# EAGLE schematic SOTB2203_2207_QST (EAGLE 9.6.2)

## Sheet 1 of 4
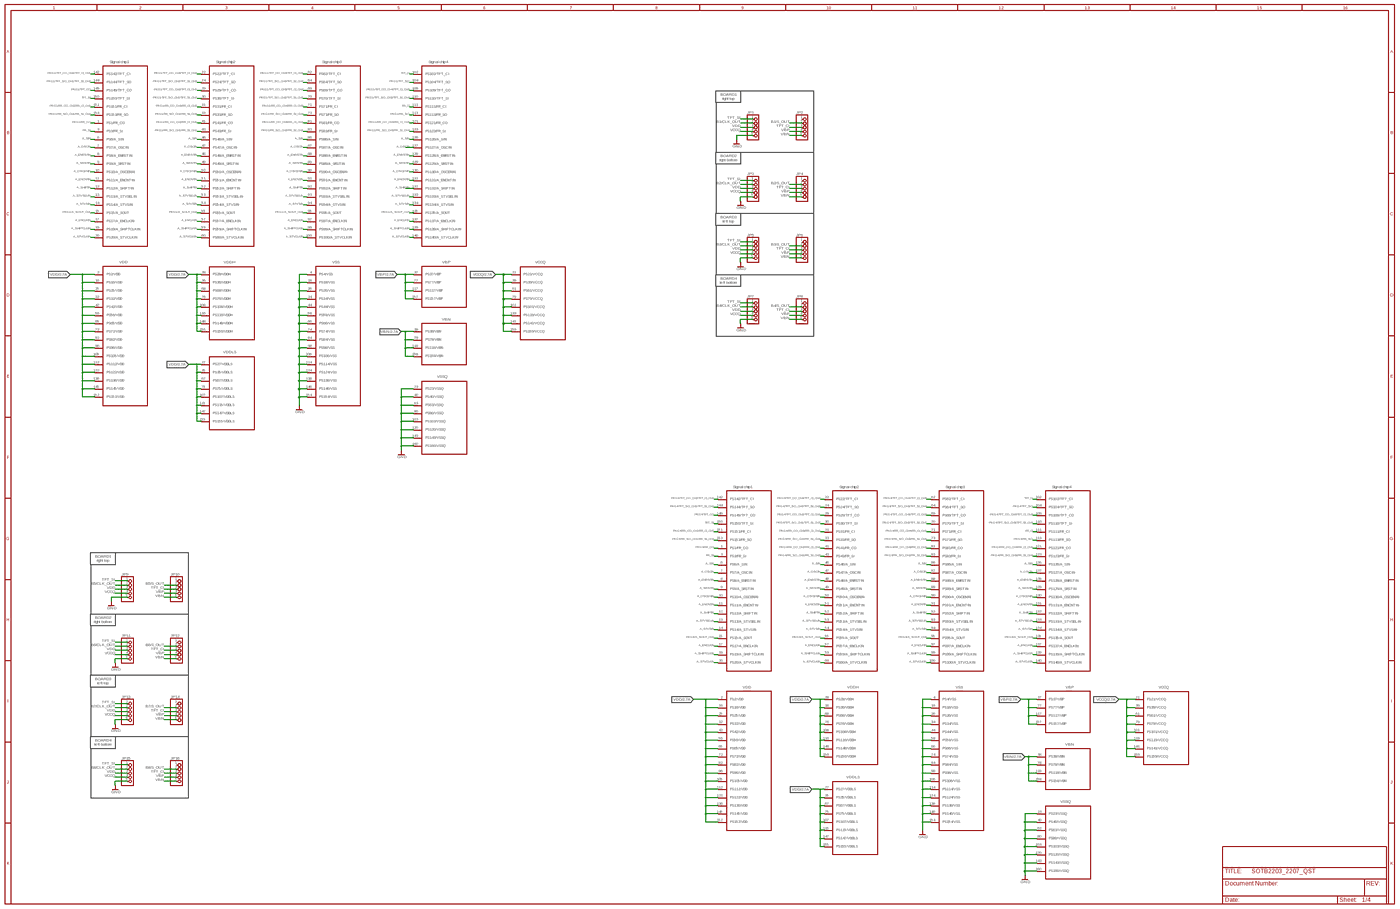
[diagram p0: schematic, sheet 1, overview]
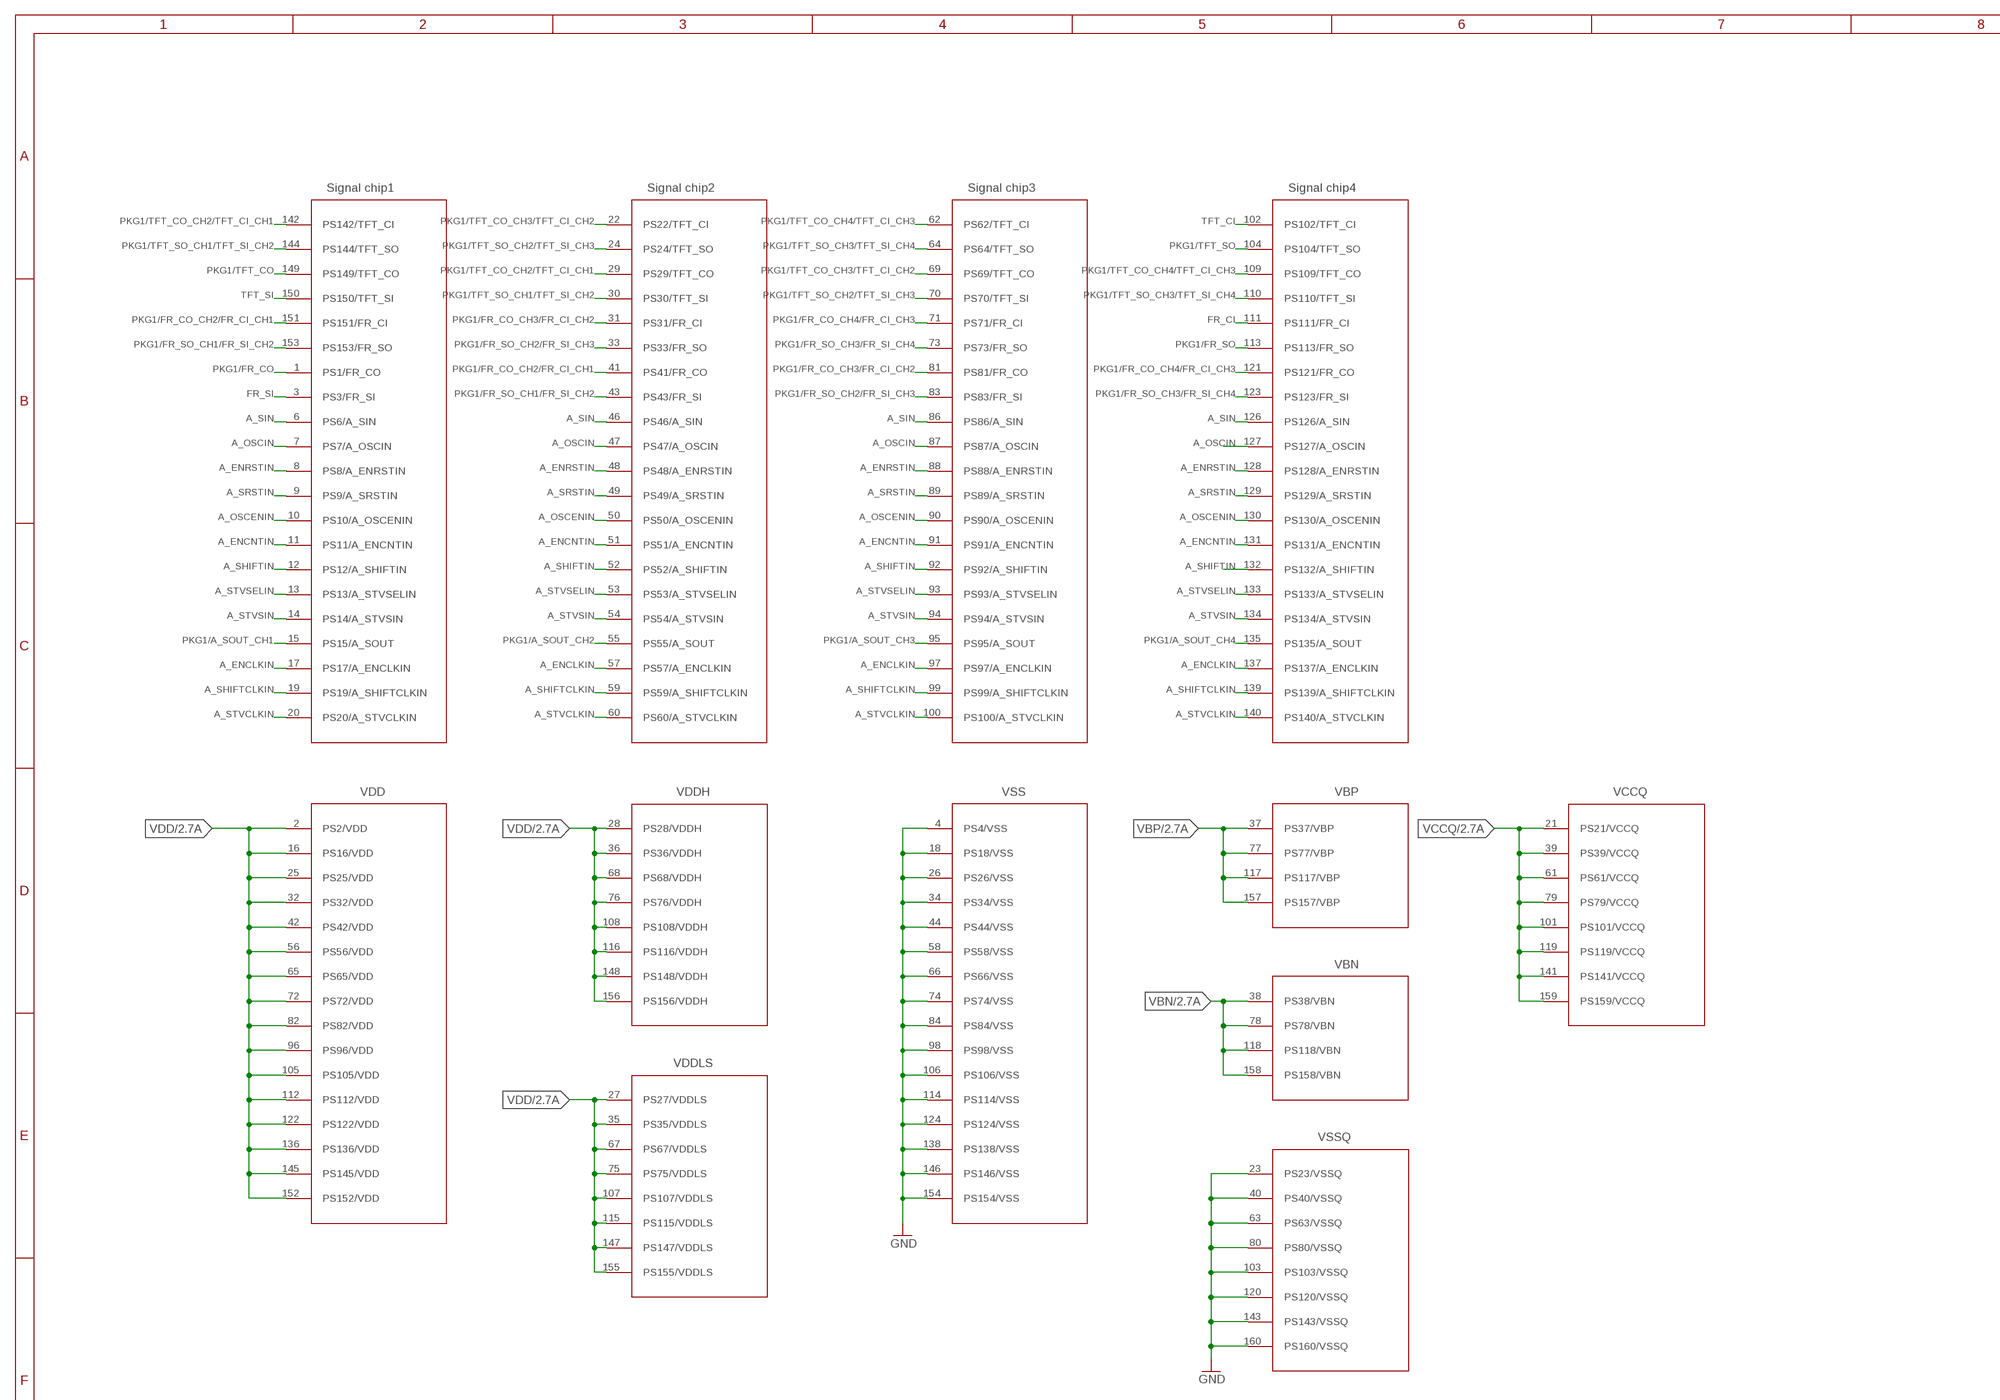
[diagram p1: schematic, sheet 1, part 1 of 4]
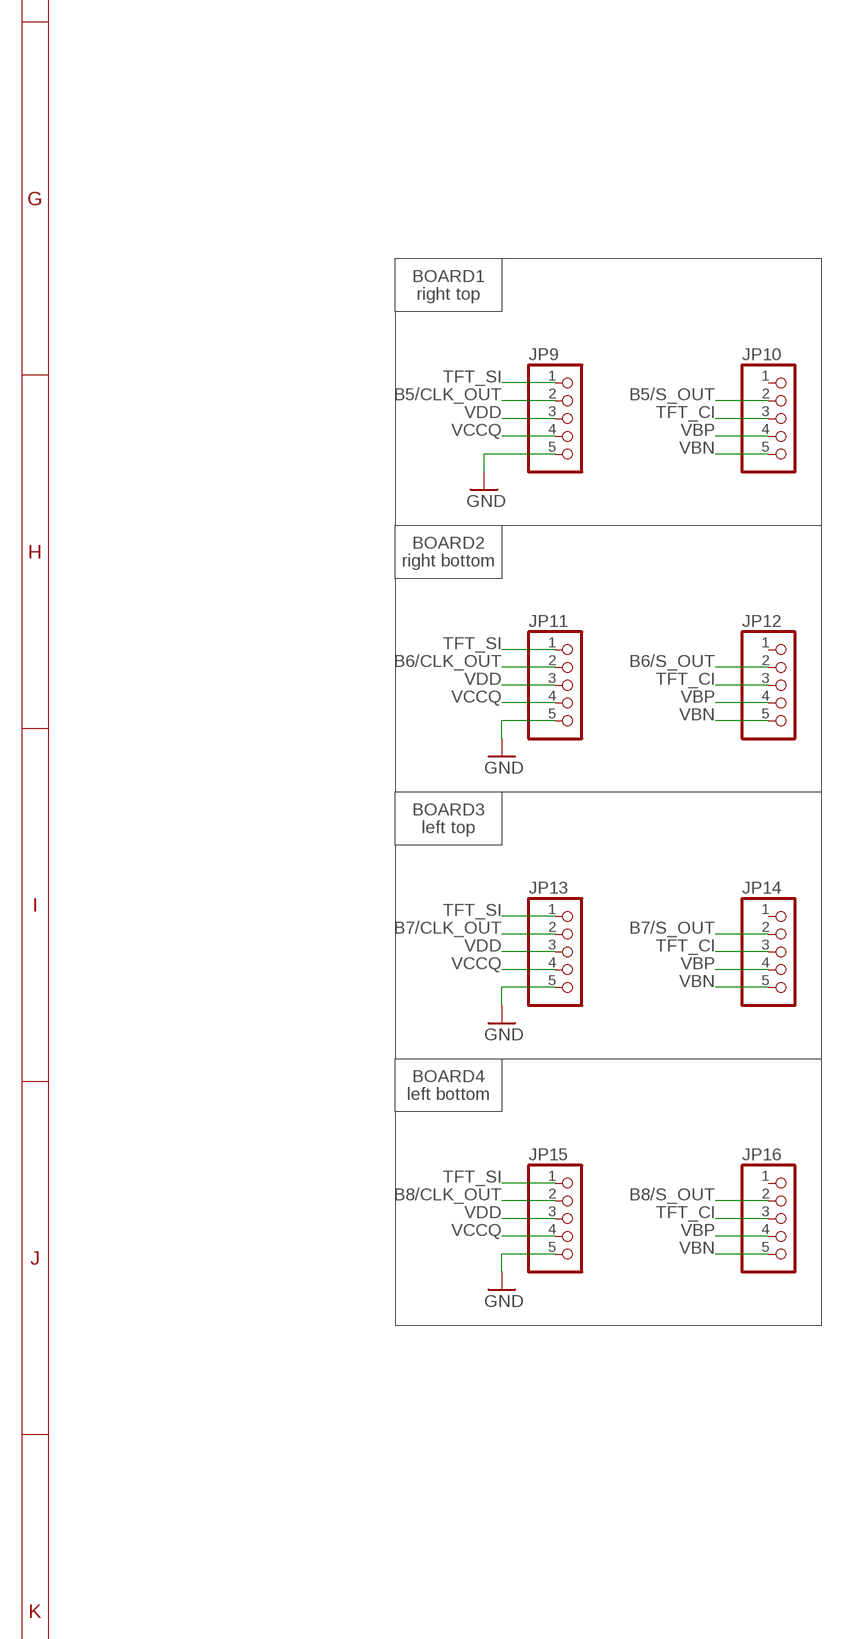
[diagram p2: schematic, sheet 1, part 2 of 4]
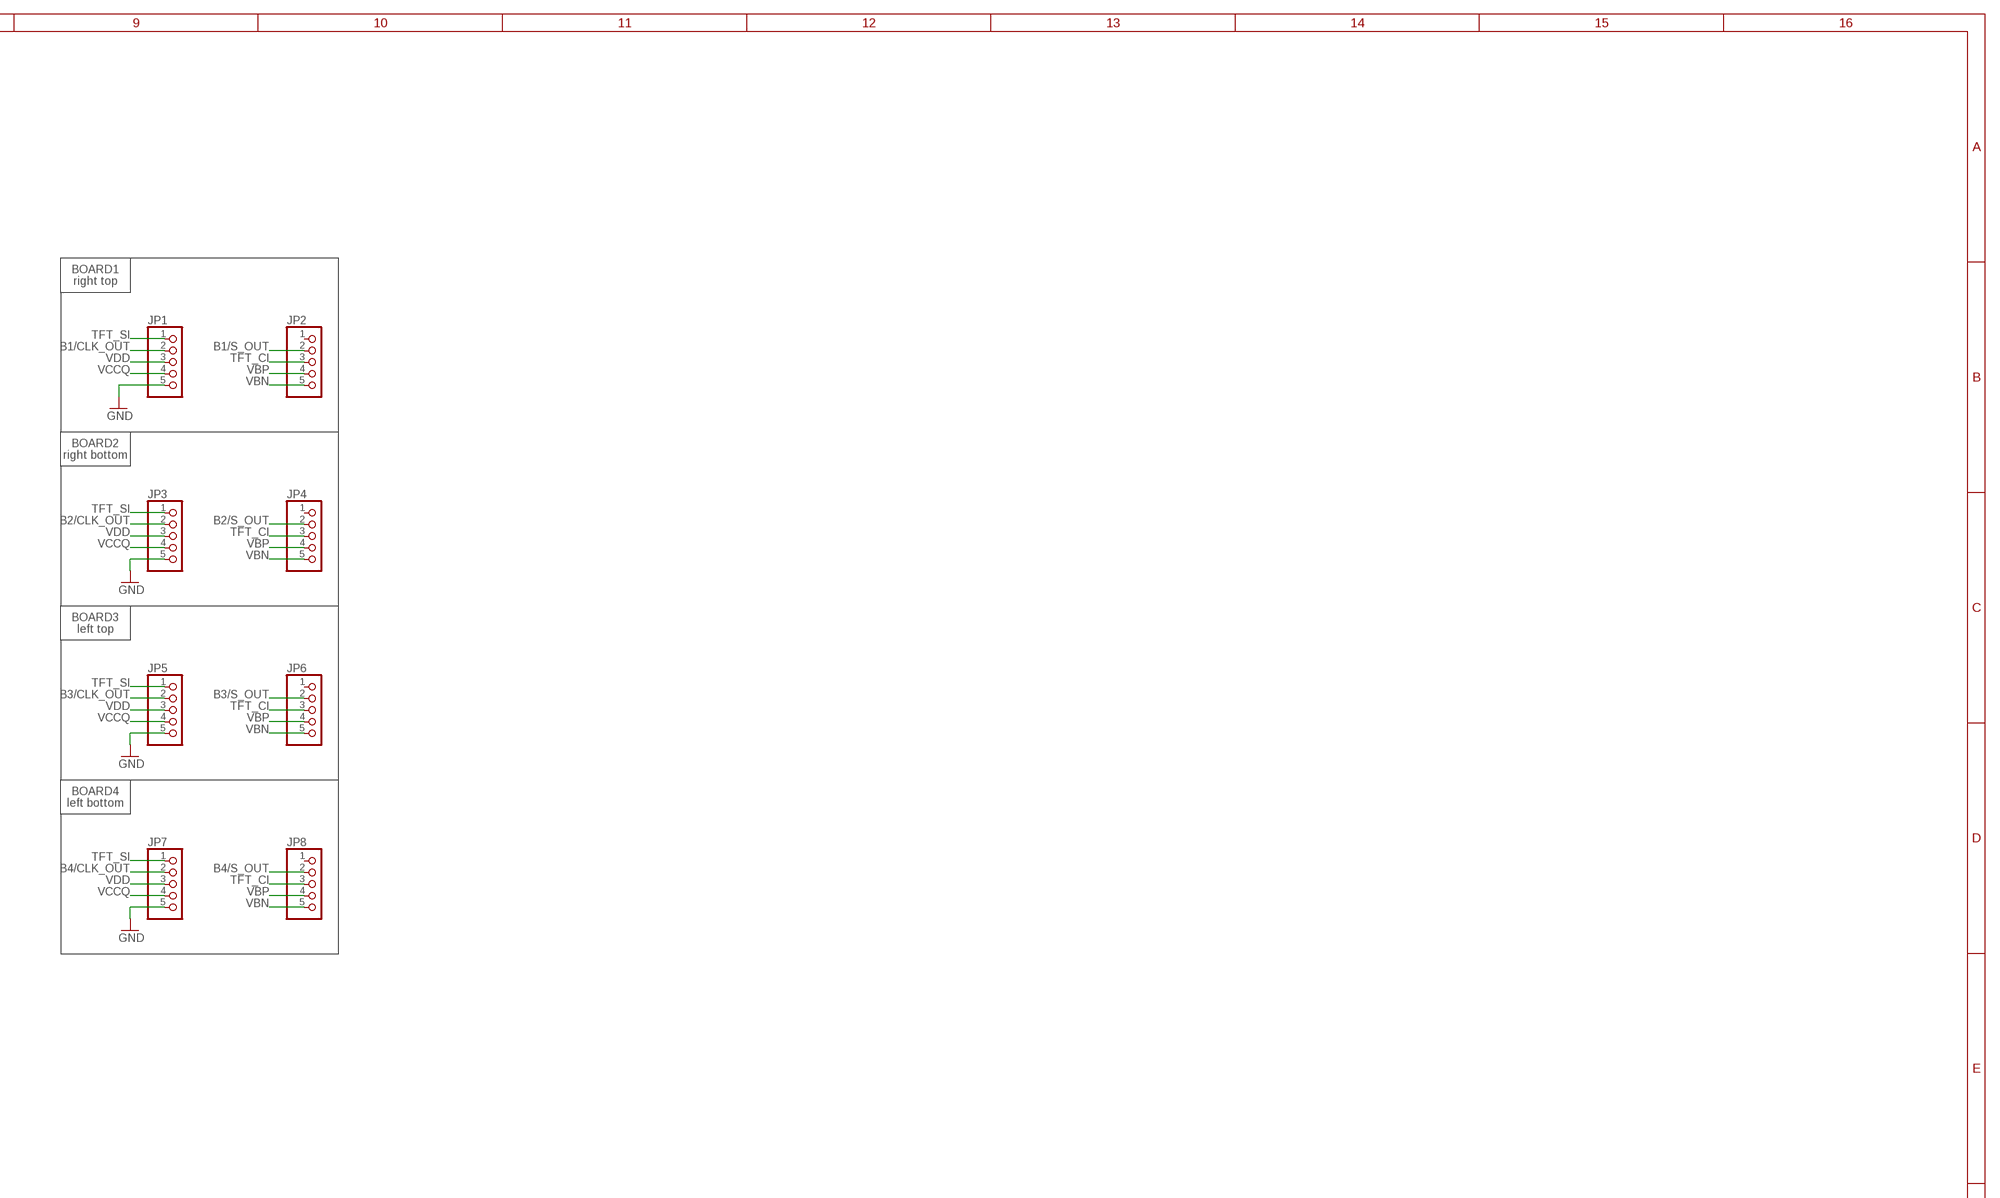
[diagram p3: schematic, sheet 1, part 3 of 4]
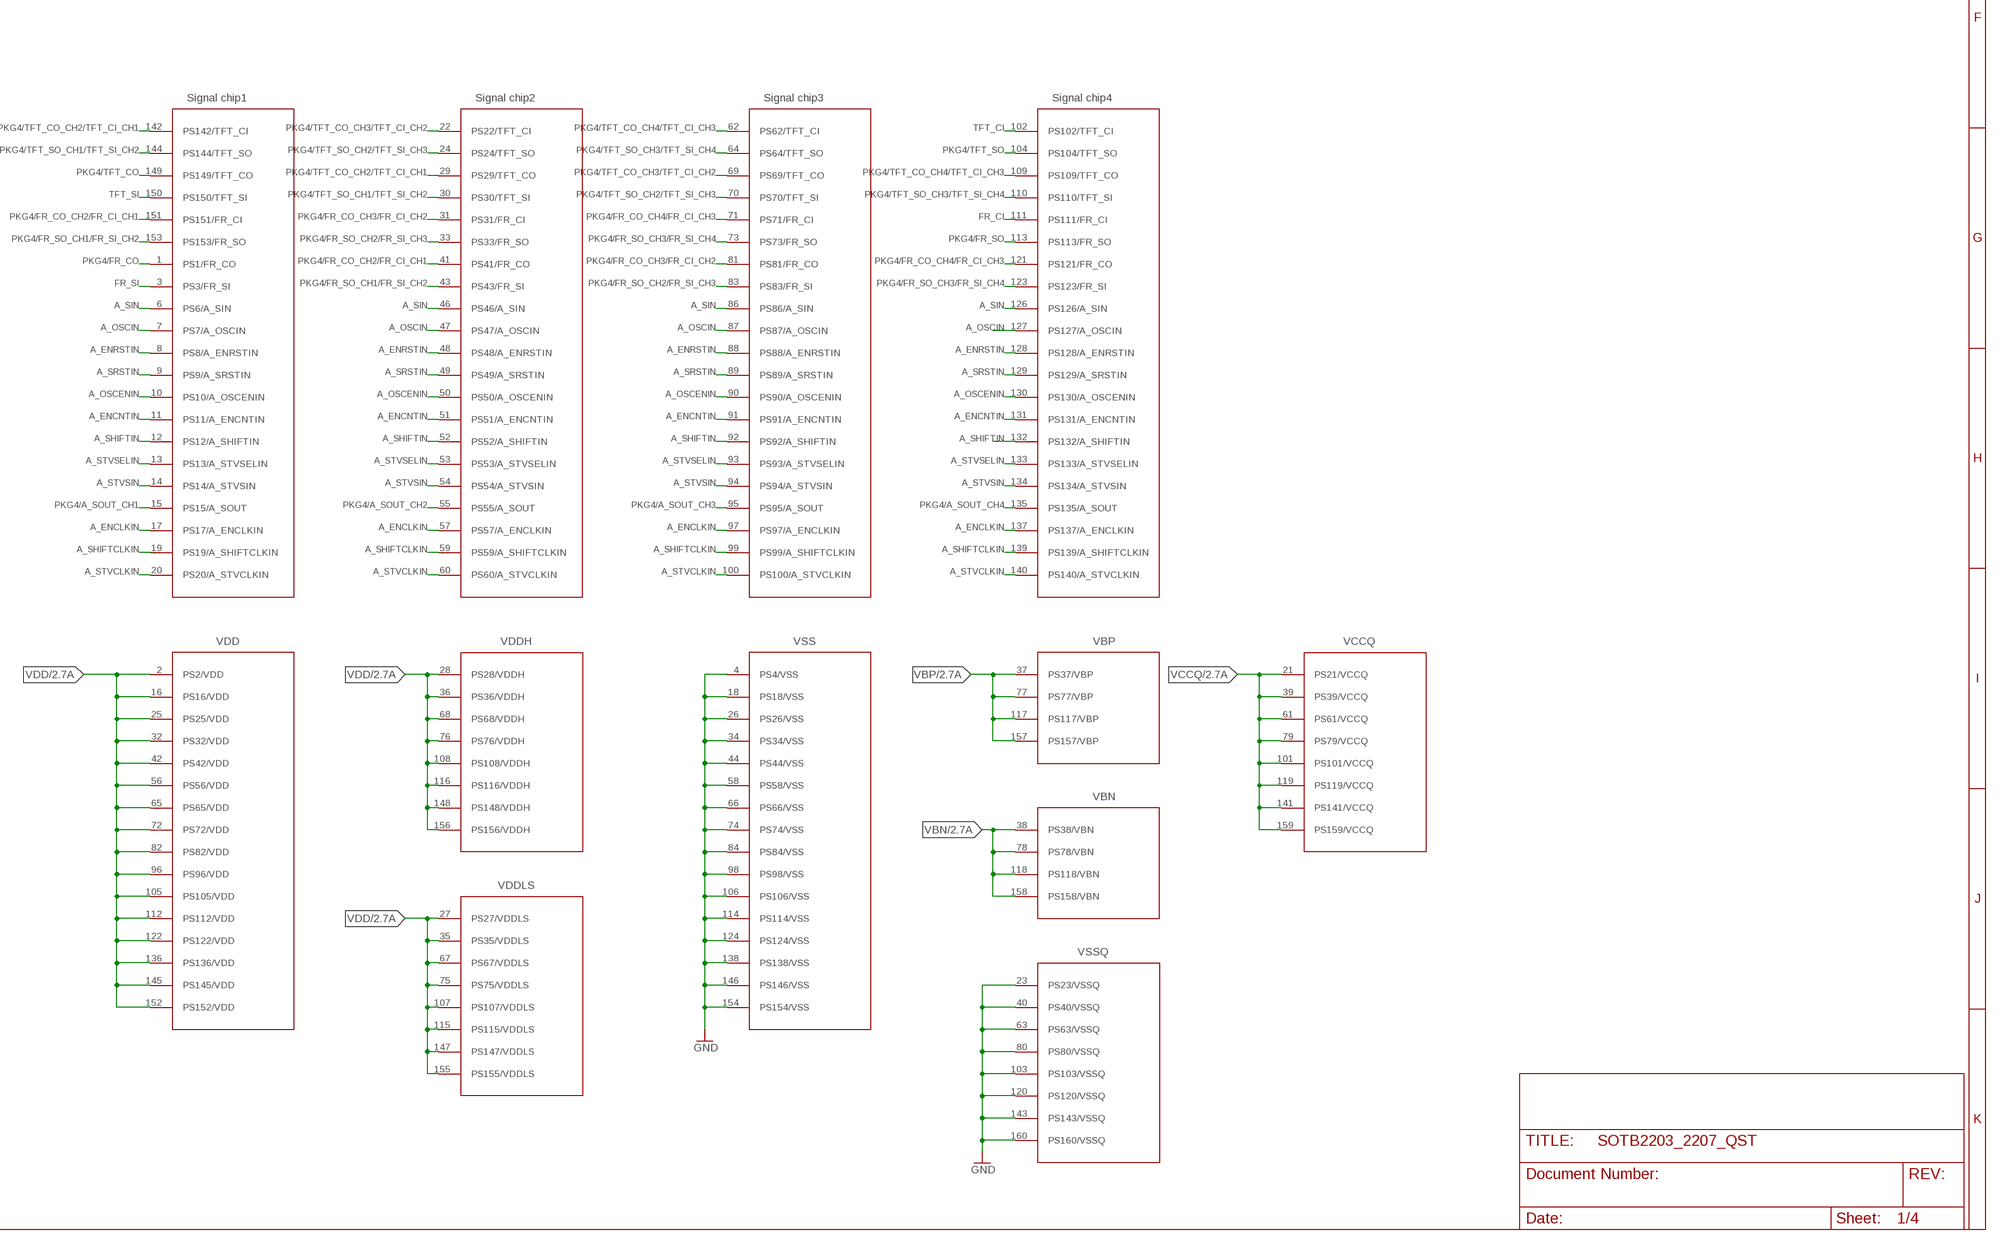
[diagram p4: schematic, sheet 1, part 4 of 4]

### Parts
JP1  PINHD-1X5  [1X05]
JP2  PINHD-1X5  [1X05]
JP3  PINHD-1X5  [1X05]
JP4  PINHD-1X5  [1X05]
JP5  PINHD-1X5  [1X05]
JP6  PINHD-1X5  [1X05]
JP7  PINHD-1X5  [1X05]
JP8  PINHD-1X5  [1X05]
JP9  PINHD-1X5  [1X05]
JP10  PINHD-1X5  [1X05]
JP11  PINHD-1X5  [1X05]
JP12  PINHD-1X5  [1X05]
JP13  PINHD-1X5  [1X05]
JP14  PINHD-1X5  [1X05]
JP15  PINHD-1X5  [1X05]
JP16  PINHD-1X5  [1X05]
PKG1  SOTB2207_4CHIP  [IC149-160-123-B5]
PKG4  SOTB2207_4CHIP  [IC149-160-123-B5]

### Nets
A_ENCLKIN: PKG1.17(PS17/A_ENCLKIN) PKG1.57(PS57/A_ENCLKIN) PKG1.97(PS97/A_ENCLKIN) PKG1.137(PS137/A_ENCLKIN) PKG4.17(PS17/A_ENCLKIN) PKG4.57(PS57/A_ENCLKIN) PKG4.97(PS97/A_ENCLKIN) PKG4.137(PS137/A_ENCLKIN) ; also sheet 2,4
A_ENCNTIN: PKG1.11(PS11/A_ENCNTIN) PKG1.51(PS51/A_ENCNTIN) PKG1.91(PS91/A_ENCNTIN) PKG1.131(PS131/A_ENCNTIN) PKG4.11(PS11/A_ENCNTIN) PKG4.51(PS51/A_ENCNTIN) PKG4.91(PS91/A_ENCNTIN) PKG4.131(PS131/A_ENCNTIN) ; also sheet 2,4
A_ENRSTIN: PKG1.8(PS8/A_ENRSTIN) PKG1.48(PS48/A_ENRSTIN) PKG1.88(PS88/A_ENRSTIN) PKG1.128(PS128/A_ENRSTIN) PKG4.8(PS8/A_ENRSTIN) PKG4.48(PS48/A_ENRSTIN) PKG4.88(PS88/A_ENRSTIN) PKG4.128(PS128/A_ENRSTIN) ; also sheet 2,4
A_OSCENIN: PKG1.10(PS10/A_OSCENIN) PKG1.50(PS50/A_OSCENIN) PKG1.90(PS90/A_OSCENIN) PKG1.130(PS130/A_OSCENIN) PKG4.10(PS10/A_OSCENIN) PKG4.50(PS50/A_OSCENIN) PKG4.90(PS90/A_OSCENIN) PKG4.130(PS130/A_OSCENIN) ; also sheet 2,4
A_OSCIN: PKG1.7(PS7/A_OSCIN) PKG1.47(PS47/A_OSCIN) PKG1.87(PS87/A_OSCIN) PKG1.127(PS127/A_OSCIN) PKG4.7(PS7/A_OSCIN) PKG4.47(PS47/A_OSCIN) PKG4.87(PS87/A_OSCIN) PKG4.127(PS127/A_OSCIN) ; also sheet 2,4
A_SHIFTCLKIN: PKG1.19(PS19/A_SHIFTCLKIN) PKG1.59(PS59/A_SHIFTCLKIN) PKG1.99(PS99/A_SHIFTCLKIN) PKG1.139(PS139/A_SHIFTCLKIN) PKG4.19(PS19/A_SHIFTCLKIN) PKG4.59(PS59/A_SHIFTCLKIN) PKG4.99(PS99/A_SHIFTCLKIN) PKG4.139(PS139/A_SHIFTCLKIN) ; also sheet 2,4
A_SHIFTIN: PKG1.12(PS12/A_SHIFTIN) PKG1.52(PS52/A_SHIFTIN) PKG1.92(PS92/A_SHIFTIN) PKG1.132(PS132/A_SHIFTIN) PKG4.12(PS12/A_SHIFTIN) PKG4.52(PS52/A_SHIFTIN) PKG4.92(PS92/A_SHIFTIN) PKG4.132(PS132/A_SHIFTIN) ; also sheet 2,4
A_SIN: PKG1.6(PS6/A_SIN) PKG1.46(PS46/A_SIN) PKG1.86(PS86/A_SIN) PKG1.126(PS126/A_SIN) PKG4.6(PS6/A_SIN) PKG4.46(PS46/A_SIN) PKG4.86(PS86/A_SIN) PKG4.126(PS126/A_SIN) ; also sheet 2,4
A_SRSTIN: PKG1.9(PS9/A_SRSTIN) PKG1.49(PS49/A_SRSTIN) PKG1.89(PS89/A_SRSTIN) PKG1.129(PS129/A_SRSTIN) PKG4.9(PS9/A_SRSTIN) PKG4.49(PS49/A_SRSTIN) PKG4.89(PS89/A_SRSTIN) PKG4.129(PS129/A_SRSTIN) ; also sheet 2,4
A_STVCLKIN: PKG1.20(PS20/A_STVCLKIN) PKG1.60(PS60/A_STVCLKIN) PKG1.100(PS100/A_STVCLKIN) PKG1.140(PS140/A_STVCLKIN) PKG4.20(PS20/A_STVCLKIN) PKG4.60(PS60/A_STVCLKIN) PKG4.100(PS100/A_STVCLKIN) PKG4.140(PS140/A_STVCLKIN) ; also sheet 2,4
A_STVSELIN: PKG1.13(PS13/A_STVSELIN) PKG1.53(PS53/A_STVSELIN) PKG1.93(PS93/A_STVSELIN) PKG1.133(PS133/A_STVSELIN) PKG4.13(PS13/A_STVSELIN) PKG4.53(PS53/A_STVSELIN) PKG4.93(PS93/A_STVSELIN) PKG4.133(PS133/A_STVSELIN) ; also sheet 2,4
A_STVSIN: PKG1.14(PS14/A_STVSIN) PKG1.54(PS54/A_STVSIN) PKG1.94(PS94/A_STVSIN) PKG1.134(PS134/A_STVSIN) PKG4.14(PS14/A_STVSIN) PKG4.54(PS54/A_STVSIN) PKG4.94(PS94/A_STVSIN) PKG4.134(PS134/A_STVSIN) ; also sheet 2,4
B1/CLK_OUT: JP1.2 ; also sheet 2,4
B1/S_OUT: JP2.2 ; also sheet 2,4
B2/CLK_OUT: JP3.2 ; also sheet 2,4
B2/S_OUT: JP4.2 ; also sheet 2,4
B3/CLK_OUT: JP5.2 ; also sheet 2,4
B3/S_OUT: JP6.2 ; also sheet 2,4
B4/CLK_OUT: JP7.2 ; also sheet 2,4
B4/S_OUT: JP8.2 ; also sheet 2,4
B5/CLK_OUT: JP9.2 ; also sheet 2,4
B5/S_OUT: JP10.2 ; also sheet 2,4
B6/CLK_OUT: JP11.2 ; also sheet 2,4
B6/S_OUT: JP12.2 ; also sheet 2,4
B7/CLK_OUT: JP13.2 ; also sheet 2,4
B7/S_OUT: JP14.2 ; also sheet 2,4
B8/CLK_OUT: JP15.2 ; also sheet 2,4
B8/S_OUT: JP16.2 ; also sheet 2,4
FR_CI: PKG1.111(PS111/FR_CI) PKG4.111(PS111/FR_CI) ; also sheet 2,4
FR_SI: PKG1.3(PS3/FR_SI) PKG4.3(PS3/FR_SI) ; also sheet 2,4
GND: JP1.5 JP3.5 JP5.5 JP7.5 JP9.5 JP11.5 JP13.5 JP15.5 PKG1.4(PS4/VSS) PKG1.18(PS18/VSS) PKG1.23(PS23/VSSQ) PKG1.26(PS26/VSS) PKG1.34(PS34/VSS) PKG1.40(PS40/VSSQ) PKG1.44(PS44/VSS) PKG1.58(PS58/VSS) PKG1.63(PS63/VSSQ) PKG1.66(PS66/VSS) PKG1.74(PS74/VSS) PKG1.80(PS80/VSSQ) PKG1.84(PS84/VSS) PKG1.98(PS98/VSS) PKG1.103(PS103/VSSQ) PKG1.106(PS106/VSS) PKG1.114(PS114/VSS) PKG1.120(PS120/VSSQ) PKG1.124(PS124/VSS) PKG1.138(PS138/VSS) PKG1.143(PS143/VSSQ) PKG1.146(PS146/VSS) PKG1.154(PS154/VSS) PKG1.160(PS160/VSSQ) PKG4.4(PS4/VSS) PKG4.18(PS18/VSS) PKG4.23(PS23/VSSQ) PKG4.26(PS26/VSS) PKG4.34(PS34/VSS) PKG4.40(PS40/VSSQ) PKG4.44(PS44/VSS) PKG4.58(PS58/VSS) PKG4.63(PS63/VSSQ) PKG4.66(PS66/VSS) PKG4.74(PS74/VSS) PKG4.80(PS80/VSSQ) PKG4.84(PS84/VSS) PKG4.98(PS98/VSS) PKG4.103(PS103/VSSQ) PKG4.106(PS106/VSS) PKG4.114(PS114/VSS) PKG4.120(PS120/VSSQ) PKG4.124(PS124/VSS) PKG4.138(PS138/VSS) PKG4.143(PS143/VSSQ) PKG4.146(PS146/VSS) PKG4.154(PS154/VSS) PKG4.160(PS160/VSSQ) ; also sheet 2,3,4
PKG1/A_SOUT_CH1: PKG1.15(PS15/A_SOUT) ; also sheet 2,4
PKG1/A_SOUT_CH2: PKG1.55(PS55/A_SOUT) ; also sheet 2,4
PKG1/A_SOUT_CH3: PKG1.95(PS95/A_SOUT) ; also sheet 2,4
PKG1/A_SOUT_CH4: PKG1.135(PS135/A_SOUT) ; also sheet 2,4
PKG1/FR_CO: PKG1.1(PS1/FR_CO) ; also sheet 2,4
PKG1/FR_CO_CH2/FR_CI_CH1: PKG1.41(PS41/FR_CO) PKG1.151(PS151/FR_CI)
PKG1/FR_CO_CH3/FR_CI_CH2: PKG1.31(PS31/FR_CI) PKG1.81(PS81/FR_CO)
PKG1/FR_CO_CH4/FR_CI_CH3: PKG1.71(PS71/FR_CI) PKG1.121(PS121/FR_CO)
PKG1/FR_SO: PKG1.113(PS113/FR_SO) ; also sheet 2,4
PKG1/FR_SO_CH1/FR_SI_CH2: PKG1.43(PS43/FR_SI) PKG1.153(PS153/FR_SO)
PKG1/FR_SO_CH2/FR_SI_CH3: PKG1.33(PS33/FR_SO) PKG1.83(PS83/FR_SI)
PKG1/FR_SO_CH3/FR_SI_CH4: PKG1.73(PS73/FR_SO) PKG1.123(PS123/FR_SI)
PKG1/TFT_CO: PKG1.149(PS149/TFT_CO) ; also sheet 2,4
PKG1/TFT_CO_CH2/TFT_CI_CH1: PKG1.29(PS29/TFT_CO) PKG1.142(PS142/TFT_CI)
PKG1/TFT_CO_CH3/TFT_CI_CH2: PKG1.22(PS22/TFT_CI) PKG1.69(PS69/TFT_CO)
PKG1/TFT_CO_CH4/TFT_CI_CH3: PKG1.62(PS62/TFT_CI) PKG1.109(PS109/TFT_CO)
PKG1/TFT_SO: PKG1.104(PS104/TFT_SO) ; also sheet 2,4
PKG1/TFT_SO_CH1/TFT_SI_CH2: PKG1.30(PS30/TFT_SI) PKG1.144(PS144/TFT_SO)
PKG1/TFT_SO_CH2/TFT_SI_CH3: PKG1.24(PS24/TFT_SO) PKG1.70(PS70/TFT_SI)
PKG1/TFT_SO_CH3/TFT_SI_CH4: PKG1.64(PS64/TFT_SO) PKG1.110(PS110/TFT_SI)
PKG4/A_SOUT_CH1: PKG4.15(PS15/A_SOUT) ; also sheet 2,4
PKG4/A_SOUT_CH2: PKG4.55(PS55/A_SOUT) ; also sheet 2,4
PKG4/A_SOUT_CH3: PKG4.95(PS95/A_SOUT) ; also sheet 2,4
PKG4/A_SOUT_CH4: PKG4.135(PS135/A_SOUT) ; also sheet 2,4
PKG4/FR_CO: PKG4.1(PS1/FR_CO) ; also sheet 2,4
PKG4/FR_CO_CH2/FR_CI_CH1: PKG4.41(PS41/FR_CO) PKG4.151(PS151/FR_CI)
PKG4/FR_CO_CH3/FR_CI_CH2: PKG4.31(PS31/FR_CI) PKG4.81(PS81/FR_CO)
PKG4/FR_CO_CH4/FR_CI_CH3: PKG4.71(PS71/FR_CI) PKG4.121(PS121/FR_CO)
PKG4/FR_SO: PKG4.113(PS113/FR_SO) ; also sheet 2,4
PKG4/FR_SO_CH1/FR_SI_CH2: PKG4.43(PS43/FR_SI) PKG4.153(PS153/FR_SO)
PKG4/FR_SO_CH2/FR_SI_CH3: PKG4.33(PS33/FR_SO) PKG4.83(PS83/FR_SI)
PKG4/FR_SO_CH3/FR_SI_CH4: PKG4.73(PS73/FR_SO) PKG4.123(PS123/FR_SI)
PKG4/TFT_CO: PKG4.149(PS149/TFT_CO) ; also sheet 2,4
PKG4/TFT_CO_CH2/TFT_CI_CH1: PKG4.29(PS29/TFT_CO) PKG4.142(PS142/TFT_CI)
PKG4/TFT_CO_CH3/TFT_CI_CH2: PKG4.22(PS22/TFT_CI) PKG4.69(PS69/TFT_CO)
PKG4/TFT_CO_CH4/TFT_CI_CH3: PKG4.62(PS62/TFT_CI) PKG4.109(PS109/TFT_CO)
PKG4/TFT_SO: PKG4.104(PS104/TFT_SO) ; also sheet 2,4
PKG4/TFT_SO_CH1/TFT_SI_CH2: PKG4.30(PS30/TFT_SI) PKG4.144(PS144/TFT_SO)
PKG4/TFT_SO_CH2/TFT_SI_CH3: PKG4.24(PS24/TFT_SO) PKG4.70(PS70/TFT_SI)
PKG4/TFT_SO_CH3/TFT_SI_CH4: PKG4.64(PS64/TFT_SO) PKG4.110(PS110/TFT_SI)
TFT_CI: JP2.3 JP4.3 JP6.3 JP8.3 JP10.3 JP12.3 JP14.3 JP16.3 PKG1.102(PS102/TFT_CI) PKG4.102(PS102/TFT_CI) ; also sheet 2,4
TFT_SI: JP1.1 JP3.1 JP5.1 JP7.1 JP9.1 JP11.1 JP13.1 JP15.1 PKG1.150(PS150/TFT_SI) PKG4.150(PS150/TFT_SI) ; also sheet 2,4
VBN: JP2.5 JP4.5 JP6.5 JP8.5 JP10.5 JP12.5 JP14.5 JP16.5 PKG1.38(PS38/VBN) PKG1.78(PS78/VBN) PKG1.118(PS118/VBN) PKG1.158(PS158/VBN) PKG4.38(PS38/VBN) PKG4.78(PS78/VBN) PKG4.118(PS118/VBN) PKG4.158(PS158/VBN) ; also sheet 2,3,4
VBP: JP2.4 JP4.4 JP6.4 JP8.4 JP10.4 JP12.4 JP14.4 JP16.4 PKG1.37(PS37/VBP) PKG1.77(PS77/VBP) PKG1.117(PS117/VBP) PKG1.157(PS157/VBP) PKG4.37(PS37/VBP) PKG4.77(PS77/VBP) PKG4.117(PS117/VBP) PKG4.157(PS157/VBP) ; also sheet 2,3,4
VCCQ: JP1.4 JP3.4 JP5.4 JP7.4 JP9.4 JP11.4 JP13.4 JP15.4 PKG1.21(PS21/VCCQ) PKG1.39(PS39/VCCQ) PKG1.61(PS61/VCCQ) PKG1.79(PS79/VCCQ) PKG1.101(PS101/VCCQ) PKG1.119(PS119/VCCQ) PKG1.141(PS141/VCCQ) PKG1.159(PS159/VCCQ) PKG4.21(PS21/VCCQ) PKG4.39(PS39/VCCQ) PKG4.61(PS61/VCCQ) PKG4.79(PS79/VCCQ) PKG4.101(PS101/VCCQ) PKG4.119(PS119/VCCQ) PKG4.141(PS141/VCCQ) PKG4.159(PS159/VCCQ) ; also sheet 2,3,4
VDD: JP1.3 JP3.3 JP5.3 JP7.3 JP9.3 JP11.3 JP13.3 JP15.3 PKG1.2(PS2/VDD) PKG1.16(PS16/VDD) PKG1.25(PS25/VDD) PKG1.27(PS27/VDDLS) PKG1.28(PS28/VDDH) PKG1.32(PS32/VDD) PKG1.35(PS35/VDDLS) PKG1.36(PS36/VDDH) PKG1.42(PS42/VDD) PKG1.56(PS56/VDD) PKG1.65(PS65/VDD) PKG1.67(PS67/VDDLS) PKG1.68(PS68/VDDH) PKG1.72(PS72/VDD) PKG1.75(PS75/VDDLS) PKG1.76(PS76/VDDH) PKG1.82(PS82/VDD) PKG1.96(PS96/VDD) PKG1.105(PS105/VDD) PKG1.107(PS107/VDDLS) PKG1.108(PS108/VDDH) PKG1.112(PS112/VDD) PKG1.115(PS115/VDDLS) PKG1.116(PS116/VDDH) PKG1.122(PS122/VDD) PKG1.136(PS136/VDD) PKG1.145(PS145/VDD) PKG1.147(PS147/VDDLS) PKG1.148(PS148/VDDH) PKG1.152(PS152/VDD) PKG1.155(PS155/VDDLS) PKG1.156(PS156/VDDH) PKG4.2(PS2/VDD) PKG4.16(PS16/VDD) PKG4.25(PS25/VDD) PKG4.27(PS27/VDDLS) PKG4.28(PS28/VDDH) PKG4.32(PS32/VDD) PKG4.35(PS35/VDDLS) PKG4.36(PS36/VDDH) PKG4.42(PS42/VDD) PKG4.56(PS56/VDD) PKG4.65(PS65/VDD) PKG4.67(PS67/VDDLS) PKG4.68(PS68/VDDH) PKG4.72(PS72/VDD) PKG4.75(PS75/VDDLS) PKG4.76(PS76/VDDH) PKG4.82(PS82/VDD) PKG4.96(PS96/VDD) PKG4.105(PS105/VDD) PKG4.107(PS107/VDDLS) PKG4.108(PS108/VDDH) PKG4.112(PS112/VDD) PKG4.115(PS115/VDDLS) PKG4.116(PS116/VDDH) PKG4.122(PS122/VDD) PKG4.136(PS136/VDD) PKG4.145(PS145/VDD) PKG4.147(PS147/VDDLS) PKG4.148(PS148/VDDH) PKG4.152(PS152/VDD) PKG4.155(PS155/VDDLS) PKG4.156(PS156/VDDH) ; also sheet 2,3,4
Unconnected: JP2.1 JP4.1 JP6.1 JP8.1 JP10.1 JP12.1 JP14.1 JP16.1

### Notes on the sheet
- BOARD1
- right top
- BOARD2
- right bottom
- BOARD3
- left top
- BOARD4
- left bottom
- BOARD1
- right top
- BOARD2
- right bottom
- BOARD3
- left top
- BOARD4
- left bottom

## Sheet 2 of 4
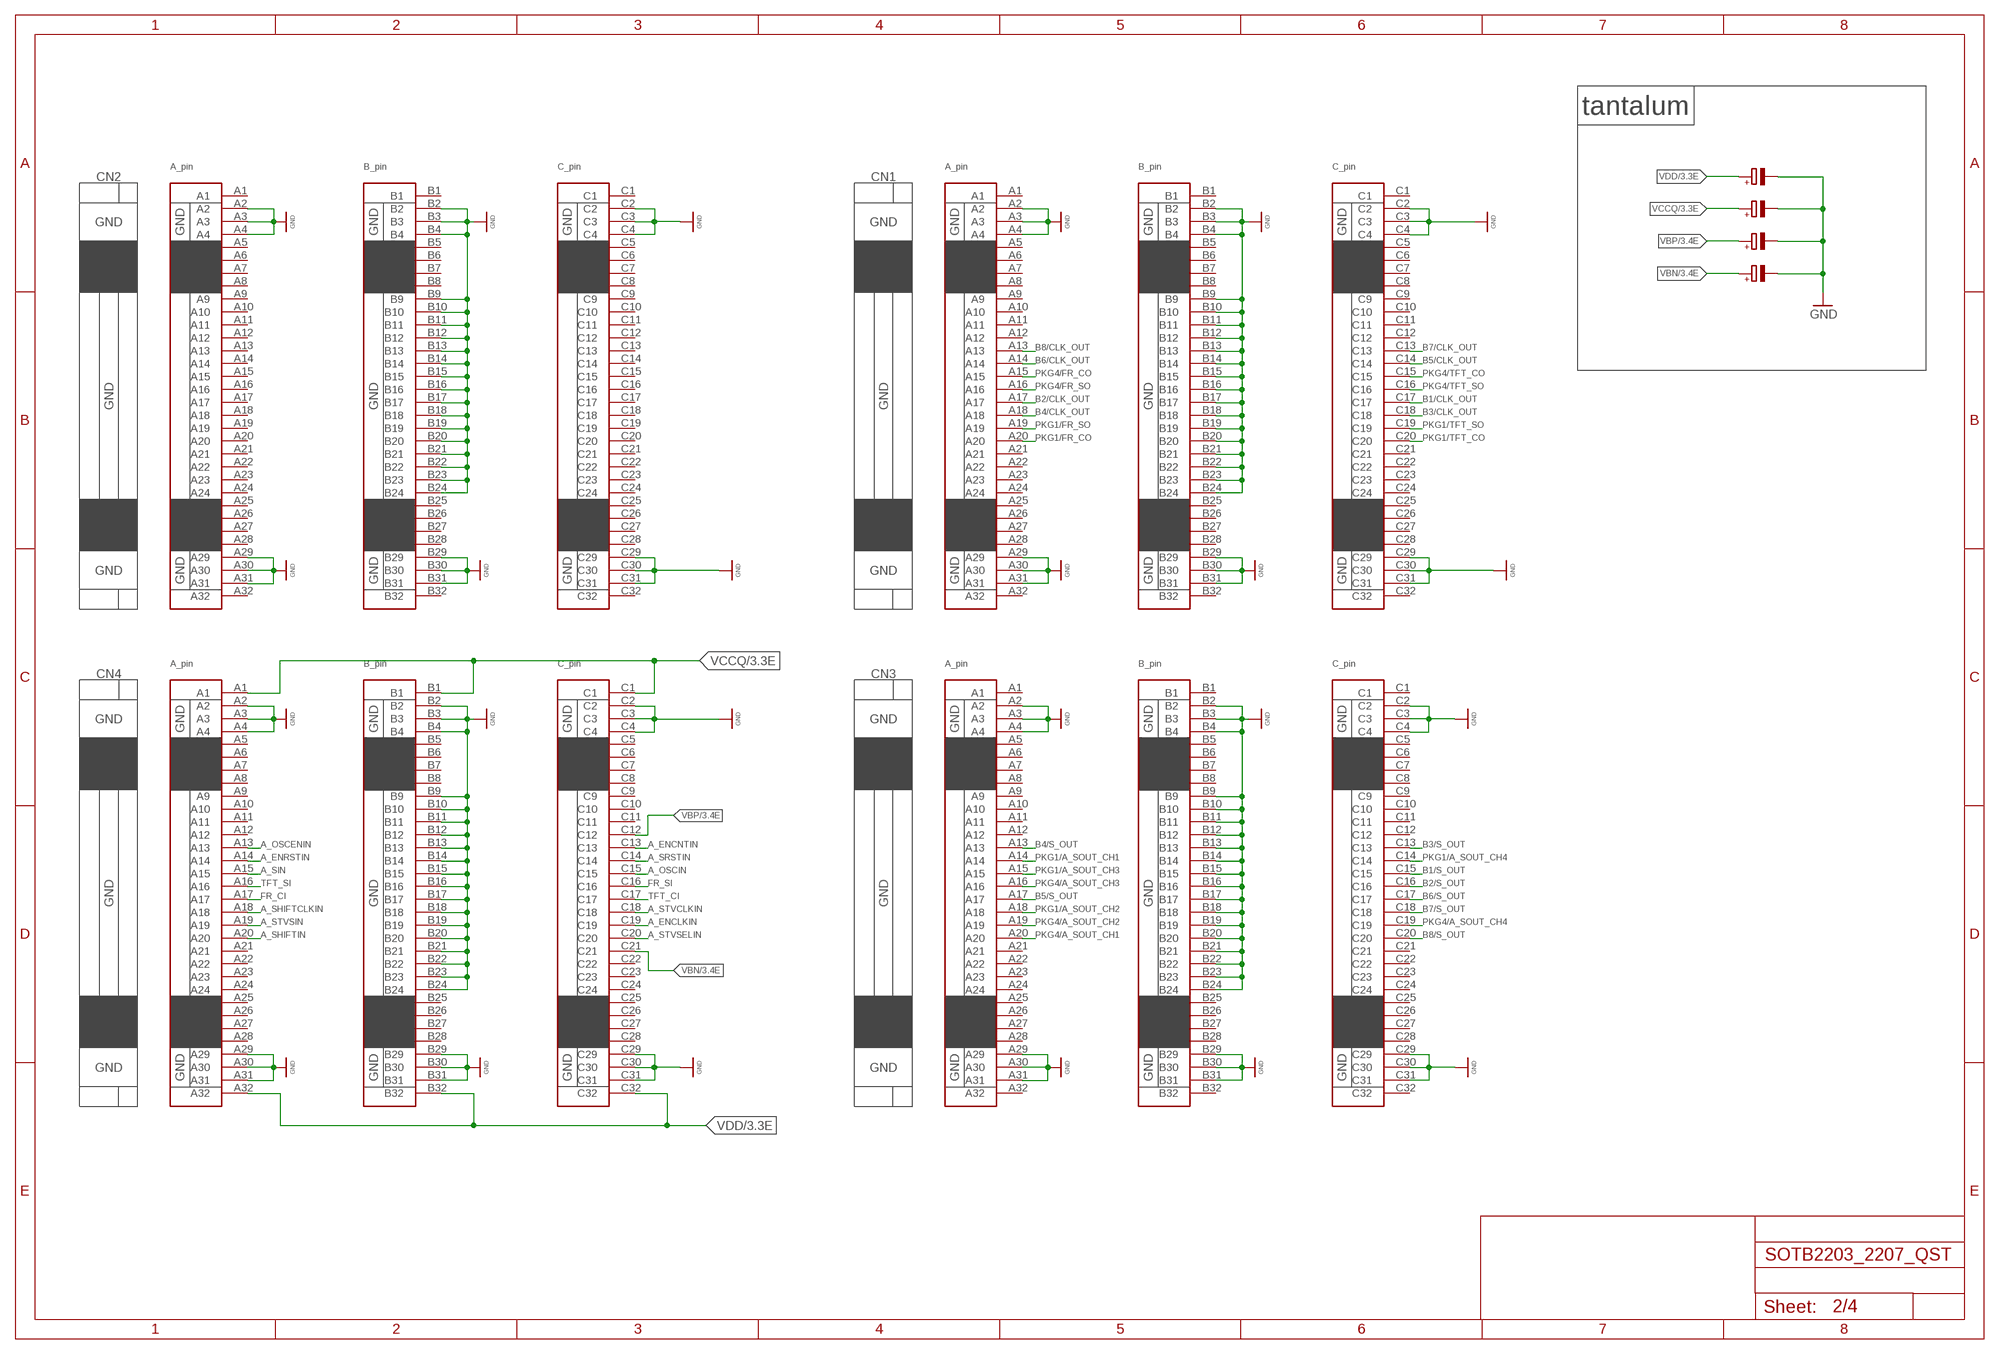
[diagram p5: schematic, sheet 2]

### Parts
CN1  XC5G-9621  [XC5D_9623]
CN2  XC5G-9621  [XC5D_9623]
CN3  XC5G-9621  [XC5D_9623]
CN4  XC5G-9621  [XC5D_9623]
U$5  TANTALUM_CAPA_F93  [6032]
U$6  TANTALUM_CAPA_F93  [6032]
U$7  TANTALUM_CAPA_F93  [6032]
U$8  TANTALUM_CAPA_F93  [6032]

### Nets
A_ENCLKIN: CN4.C19 ; also sheet 1,4
A_ENCNTIN: CN4.C13 ; also sheet 1,4
A_ENRSTIN: CN4.A14 ; also sheet 1,4
A_OSCENIN: CN4.A13 ; also sheet 1,4
A_OSCIN: CN4.C15 ; also sheet 1,4
A_SHIFTCLKIN: CN4.A18 ; also sheet 1,4
A_SHIFTIN: CN4.A20 ; also sheet 1,4
A_SIN: CN4.A15 ; also sheet 1,4
A_SRSTIN: CN4.C14 ; also sheet 1,4
A_STVCLKIN: CN4.C18 ; also sheet 1,4
A_STVSELIN: CN4.C20 ; also sheet 1,4
A_STVSIN: CN4.A19 ; also sheet 1,4
B1/CLK_OUT: CN1.C17 ; also sheet 1,4
B1/S_OUT: CN3.C15 ; also sheet 1,4
B2/CLK_OUT: CN1.A17 ; also sheet 1,4
B2/S_OUT: CN3.C16 ; also sheet 1,4
B3/CLK_OUT: CN1.C18 ; also sheet 1,4
B3/S_OUT: CN3.C13 ; also sheet 1,4
B4/CLK_OUT: CN1.A18 ; also sheet 1,4
B4/S_OUT: CN3.A13 ; also sheet 1,4
B5/CLK_OUT: CN1.C14 ; also sheet 1,4
B5/S_OUT: CN3.A17 ; also sheet 1,4
B6/CLK_OUT: CN1.A14 ; also sheet 1,4
B6/S_OUT: CN3.C17 ; also sheet 1,4
B7/CLK_OUT: CN1.C13 ; also sheet 1,4
B7/S_OUT: CN3.C18 ; also sheet 1,4
B8/CLK_OUT: CN1.A13 ; also sheet 1,4
B8/S_OUT: CN3.C20 ; also sheet 1,4
FR_CI: CN4.A17 ; also sheet 1,4
FR_SI: CN4.C16 ; also sheet 1,4
GND: CN1.A2 CN1.A3 CN1.A4 CN1.A29 CN1.A30 CN1.A31 CN1.B2 CN1.B3 CN1.B4 CN1.B9 CN1.B10 CN1.B11 CN1.B12 CN1.B13 CN1.B14 CN1.B15 CN1.B16 CN1.B17 CN1.B18 CN1.B19 CN1.B20 CN1.B21 CN1.B22 CN1.B23 CN1.B24 CN1.B29 CN1.B30 CN1.B31 CN1.C2 CN1.C3 CN1.C4 CN1.C29 CN1.C30 CN1.C31 CN2.A2 CN2.A3 CN2.A4 CN2.A29 CN2.A30 CN2.A31 CN2.B2 CN2.B3 CN2.B4 CN2.B9 CN2.B10 CN2.B11 CN2.B12 CN2.B13 CN2.B14 CN2.B15 CN2.B16 CN2.B17 CN2.B18 CN2.B19 CN2.B20 CN2.B21 CN2.B22 CN2.B23 CN2.B24 CN2.B29 CN2.B30 CN2.B31 CN2.C2 CN2.C3 CN2.C4 CN2.C29 CN2.C30 CN2.C31 CN3.A2 CN3.A3 CN3.A4 CN3.A29 CN3.A30 CN3.A31 CN3.B2 CN3.B3 CN3.B4 CN3.B9 CN3.B10 CN3.B11 CN3.B12 CN3.B13 CN3.B14 CN3.B15 CN3.B16 CN3.B17 CN3.B18 CN3.B19 CN3.B20 CN3.B21 CN3.B22 CN3.B23 CN3.B24 CN3.B29 CN3.B30 CN3.B31 CN3.C2 CN3.C3 CN3.C4 CN3.C29 CN3.C30 CN3.C31 CN4.A2 CN4.A3 CN4.A4 CN4.A29 CN4.A30 CN4.A31 CN4.B2 CN4.B3 CN4.B4 CN4.B9 CN4.B10 CN4.B11 CN4.B12 CN4.B13 CN4.B14 CN4.B15 CN4.B16 CN4.B17 CN4.B18 CN4.B19 CN4.B20 CN4.B21 CN4.B22 CN4.B23 CN4.B24 CN4.B29 CN4.B30 CN4.B31 CN4.C2 CN4.C3 CN4.C4 CN4.C29 CN4.C30 CN4.C31 U$5.- U$6.- U$7.- U$8.- ; also sheet 1,3,4
PKG1/A_SOUT_CH1: CN3.A14 ; also sheet 1,4
PKG1/A_SOUT_CH2: CN3.A18 ; also sheet 1,4
PKG1/A_SOUT_CH3: CN3.A15 ; also sheet 1,4
PKG1/A_SOUT_CH4: CN3.C14 ; also sheet 1,4
PKG1/FR_CO: CN1.A20 ; also sheet 1,4
PKG1/FR_SO: CN1.A19 ; also sheet 1,4
PKG1/TFT_CO: CN1.C20 ; also sheet 1,4
PKG1/TFT_SO: CN1.C19 ; also sheet 1,4
PKG4/A_SOUT_CH1: CN3.A20 ; also sheet 1,4
PKG4/A_SOUT_CH2: CN3.A19 ; also sheet 1,4
PKG4/A_SOUT_CH3: CN3.A16 ; also sheet 1,4
PKG4/A_SOUT_CH4: CN3.C19 ; also sheet 1,4
PKG4/FR_CO: CN1.A15 ; also sheet 1,4
PKG4/FR_SO: CN1.A16 ; also sheet 1,4
PKG4/TFT_CO: CN1.C15 ; also sheet 1,4
PKG4/TFT_SO: CN1.C16 ; also sheet 1,4
TFT_CI: CN4.C17 ; also sheet 1,4
TFT_SI: CN4.A16 ; also sheet 1,4
VBN: CN4.C21 U$8.+ ; also sheet 1,3,4
VBP: CN4.C12 U$7.+ ; also sheet 1,3,4
VCCQ: CN4.A1 CN4.B1 CN4.C1 U$6.+ ; also sheet 1,3,4
VDD: CN4.A32 CN4.B32 CN4.C32 U$5.+ ; also sheet 1,3,4
Unconnected: CN1.A1 CN1.A5 CN1.A6 CN1.A7 CN1.A8 CN1.A9 CN1.A10 CN1.A11 CN1.A12 CN1.A21 CN1.A22 CN1.A23 CN1.A24 CN1.A25 CN1.A26 CN1.A27 CN1.A28 CN1.A32 CN1.B1 CN1.B5 CN1.B6 CN1.B7 CN1.B8 CN1.B25 CN1.B26 CN1.B27 CN1.B28 CN1.B32 CN1.C1 CN1.C5 CN1.C6 CN1.C7 CN1.C8 CN1.C9 CN1.C10 CN1.C11 CN1.C12 CN1.C21 CN1.C22 CN1.C23 CN1.C24 CN1.C25 CN1.C26 CN1.C27 CN1.C28 CN1.C32 CN2.A1 CN2.A5 CN2.A6 CN2.A7 CN2.A8 CN2.A9 CN2.A10 CN2.A11 CN2.A12 CN2.A13 CN2.A14 CN2.A15 CN2.A16 CN2.A17 CN2.A18 CN2.A19 CN2.A20 CN2.A21 CN2.A22 CN2.A23 CN2.A24 CN2.A25 CN2.A26 CN2.A27 CN2.A28 CN2.A32 CN2.B1 CN2.B5 CN2.B6 CN2.B7 CN2.B8 CN2.B25 CN2.B26 CN2.B27 CN2.B28 CN2.B32 CN2.C1 CN2.C5 CN2.C6 CN2.C7 CN2.C8 CN2.C9 CN2.C10 CN2.C11 CN2.C12 CN2.C13 CN2.C14 CN2.C15 CN2.C16 CN2.C17 CN2.C18 CN2.C19 CN2.C20 CN2.C21 CN2.C22 CN2.C23 CN2.C24 CN2.C25 CN2.C26 CN2.C27 CN2.C28 CN2.C32 CN3.A1 CN3.A5 CN3.A6 CN3.A7 CN3.A8 CN3.A9 CN3.A10 CN3.A11 CN3.A12 CN3.A21 CN3.A22 CN3.A23 CN3.A24 CN3.A25 CN3.A26 CN3.A27 CN3.A28 CN3.A32 CN3.B1 CN3.B5 CN3.B6 CN3.B7 CN3.B8 CN3.B25 CN3.B26 CN3.B27 CN3.B28 CN3.B32 CN3.C1 CN3.C5 CN3.C6 CN3.C7 CN3.C8 CN3.C9 CN3.C10 CN3.C11 CN3.C12 CN3.C21 CN3.C22 CN3.C23 CN3.C24 CN3.C25 CN3.C26 CN3.C27 CN3.C28 CN3.C32 CN4.A5 CN4.A6 CN4.A7 CN4.A8 CN4.A9 CN4.A10 CN4.A11 CN4.A12 CN4.A21 CN4.A22 CN4.A23 CN4.A24 CN4.A25 CN4.A26 CN4.A27 CN4.A28 CN4.B5 CN4.B6 CN4.B7 CN4.B8 CN4.B25 CN4.B26 CN4.B27 CN4.B28 CN4.C5 CN4.C6 CN4.C7 CN4.C8 CN4.C9 CN4.C10 CN4.C11 CN4.C22 CN4.C23 CN4.C24 CN4.C25 CN4.C26 CN4.C27 CN4.C28

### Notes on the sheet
- tantalum
- CN2 | CN1
- GND | GND | GND | GND | GND | GND | GND | GND
- GND | GND | GND | GND
- GND | GND | GND | GND | GND | GND | GND | GND
- CN4 | CN3
- GND | GND | GND | GND | GND | GND | GND | GND
- GND | GND | GND | GND
- GND | GND | GND | GND | GND | GND | GND | GND

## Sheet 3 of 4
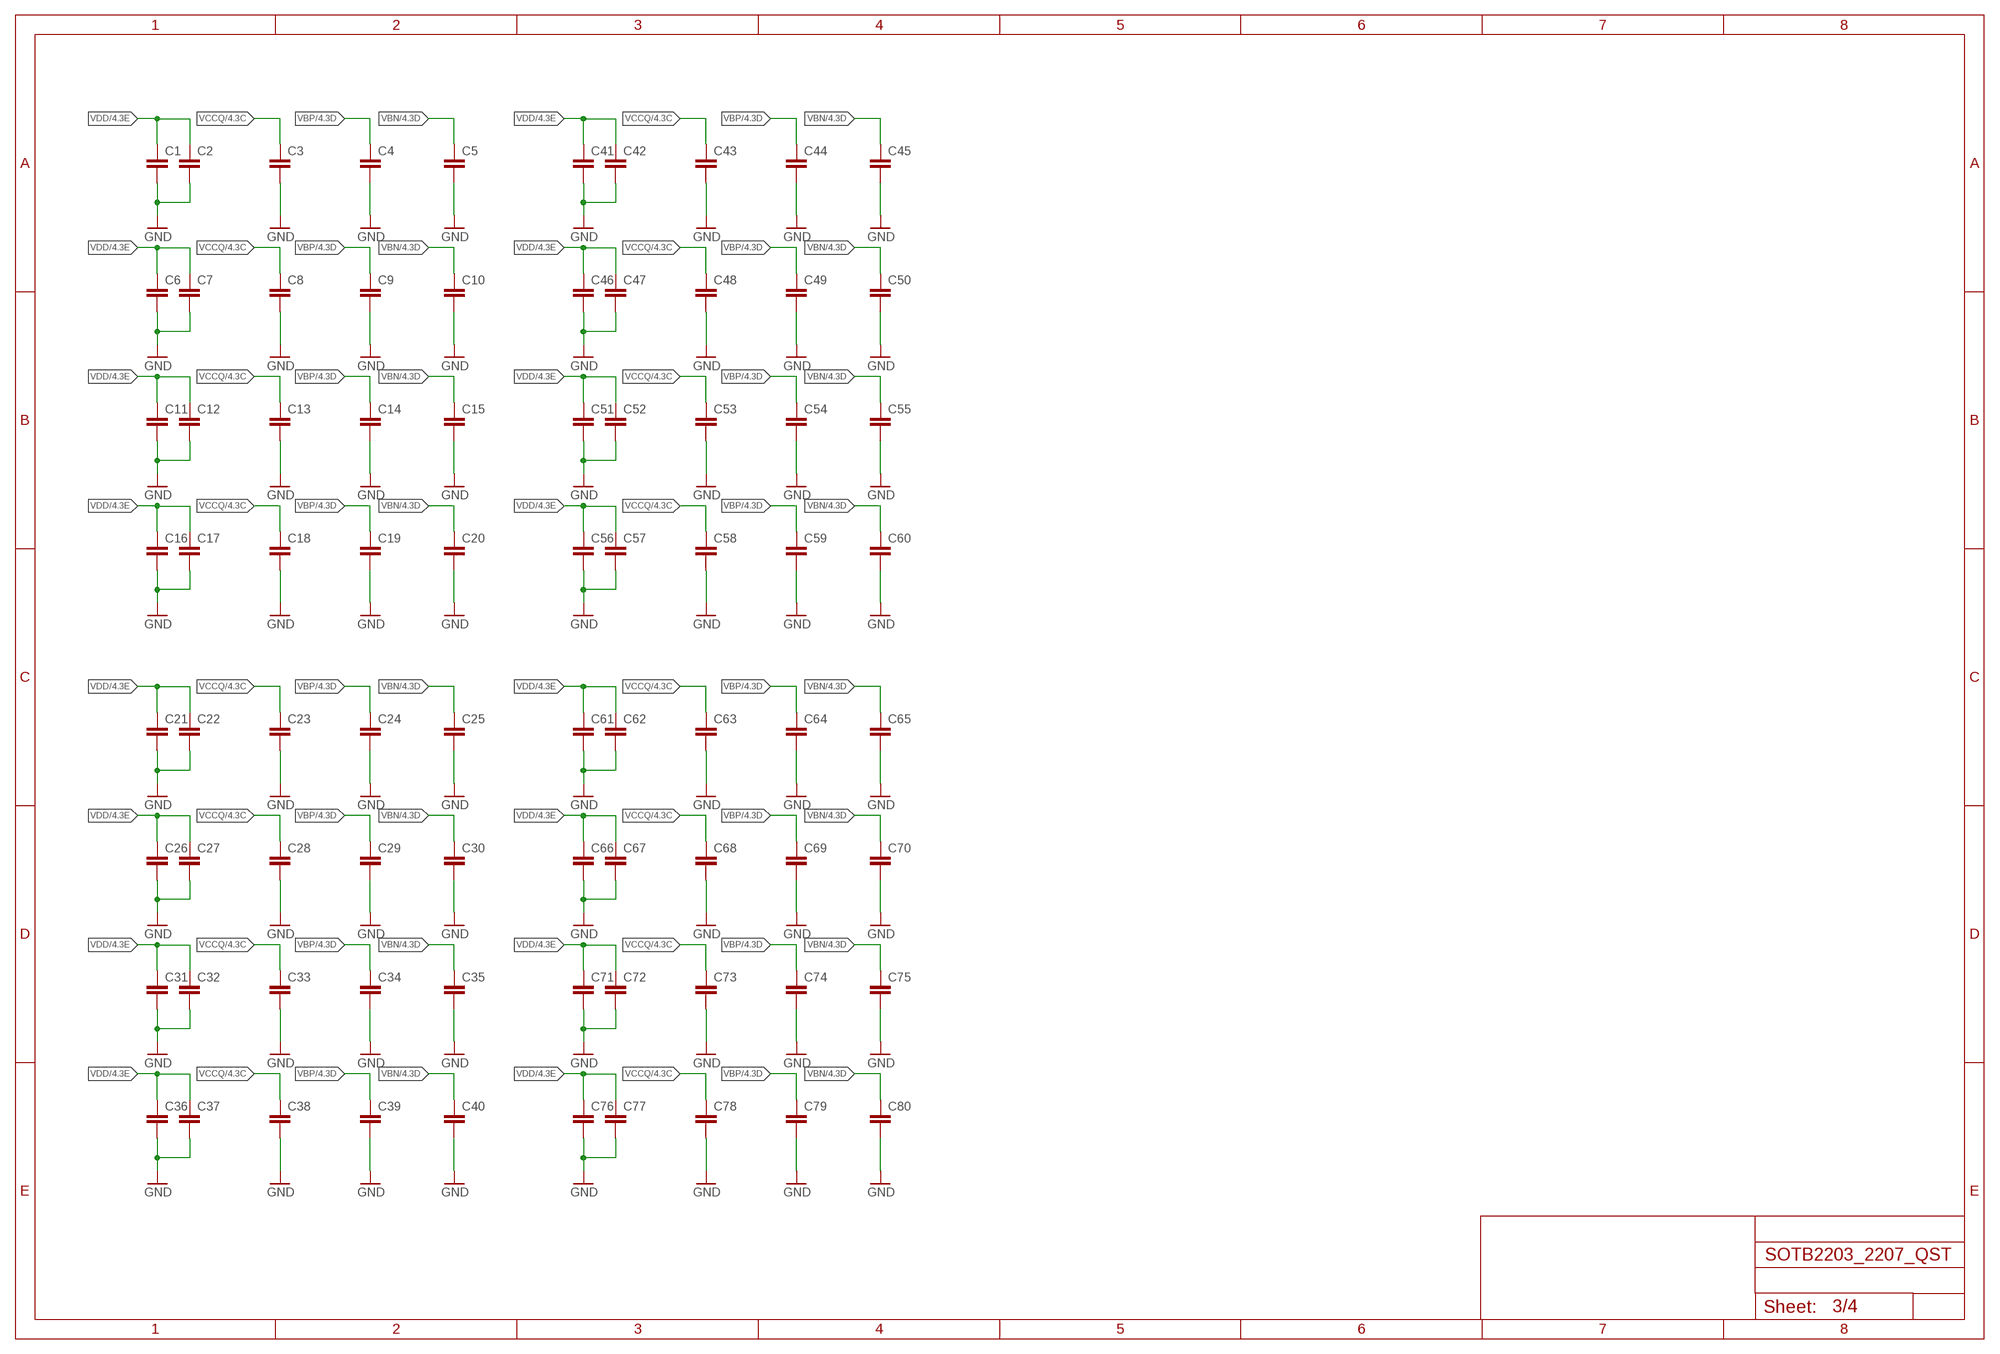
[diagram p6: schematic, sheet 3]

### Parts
C1  C-EUC0603K  [C0603K]
C2  C-EUC0603K  [C0603K]
C3  C-EUC0603K  [C0603K]
C4  C-EUC0603K  [C0603K]
C5  C-EUC0603K  [C0603K]
C6  C-EUC0603K  [C0603K]
C7  C-EUC0603K  [C0603K]
C8  C-EUC0603K  [C0603K]
C9  C-EUC0603K  [C0603K]
C10  C-EUC0603K  [C0603K]
C11  C-EUC0603K  [C0603K]
C12  C-EUC0603K  [C0603K]
C13  C-EUC0603K  [C0603K]
C14  C-EUC0603K  [C0603K]
C15  C-EUC0603K  [C0603K]
C16  C-EUC0603K  [C0603K]
C17  C-EUC0603K  [C0603K]
C18  C-EUC0603K  [C0603K]
C19  C-EUC0603K  [C0603K]
C20  C-EUC0603K  [C0603K]
C21  C-EUC0603K  [C0603K]
C22  C-EUC0603K  [C0603K]
C23  C-EUC0603K  [C0603K]
C24  C-EUC0603K  [C0603K]
C25  C-EUC0603K  [C0603K]
C26  C-EUC0603K  [C0603K]
C27  C-EUC0603K  [C0603K]
C28  C-EUC0603K  [C0603K]
C29  C-EUC0603K  [C0603K]
C30  C-EUC0603K  [C0603K]
C31  C-EUC0603K  [C0603K]
C32  C-EUC0603K  [C0603K]
C33  C-EUC0603K  [C0603K]
C34  C-EUC0603K  [C0603K]
C35  C-EUC0603K  [C0603K]
C36  C-EUC0603K  [C0603K]
C37  C-EUC0603K  [C0603K]
C38  C-EUC0603K  [C0603K]
C39  C-EUC0603K  [C0603K]
C40  C-EUC0603K  [C0603K]
C41  C-EUC0603K  [C0603K]
C42  C-EUC0603K  [C0603K]
C43  C-EUC0603K  [C0603K]
C44  C-EUC0603K  [C0603K]
C45  C-EUC0603K  [C0603K]
C46  C-EUC0603K  [C0603K]
C47  C-EUC0603K  [C0603K]
C48  C-EUC0603K  [C0603K]
C49  C-EUC0603K  [C0603K]
C50  C-EUC0603K  [C0603K]
C51  C-EUC0603K  [C0603K]
C52  C-EUC0603K  [C0603K]
C53  C-EUC0603K  [C0603K]
C54  C-EUC0603K  [C0603K]
C55  C-EUC0603K  [C0603K]
C56  C-EUC0603K  [C0603K]
C57  C-EUC0603K  [C0603K]
C58  C-EUC0603K  [C0603K]
C59  C-EUC0603K  [C0603K]
C60  C-EUC0603K  [C0603K]
C61  C-EUC0603K  [C0603K]
C62  C-EUC0603K  [C0603K]
C63  C-EUC0603K  [C0603K]
C64  C-EUC0603K  [C0603K]
C65  C-EUC0603K  [C0603K]
C66  C-EUC0603K  [C0603K]
C67  C-EUC0603K  [C0603K]
C68  C-EUC0603K  [C0603K]
C69  C-EUC0603K  [C0603K]
C70  C-EUC0603K  [C0603K]
C71  C-EUC0603K  [C0603K]
C72  C-EUC0603K  [C0603K]
C73  C-EUC0603K  [C0603K]
C74  C-EUC0603K  [C0603K]
C75  C-EUC0603K  [C0603K]
C76  C-EUC0603K  [C0603K]
C77  C-EUC0603K  [C0603K]
C78  C-EUC0603K  [C0603K]
C79  C-EUC0603K  [C0603K]
C80  C-EUC0603K  [C0603K]

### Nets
GND: C1.2 C2.2 C3.2 C4.2 C5.2 C6.2 C7.2 C8.2 C9.2 C10.2 C11.2 C12.2 C13.2 C14.2 C15.2 C16.2 C17.2 C18.2 C19.2 C20.2 C21.2 C22.2 C23.2 C24.2 C25.2 C26.2 C27.2 C28.2 C29.2 C30.2 C31.2 C32.2 C33.2 C34.2 C35.2 C36.2 C37.2 C38.2 C39.2 C40.2 C41.2 C42.2 C43.2 C44.2 C45.2 C46.2 C47.2 C48.2 C49.2 C50.2 C51.2 C52.2 C53.2 C54.2 C55.2 C56.2 C57.2 C58.2 C59.2 C60.2 C61.2 C62.2 C63.2 C64.2 C65.2 C66.2 C67.2 C68.2 C69.2 C70.2 C71.2 C72.2 C73.2 C74.2 C75.2 C76.2 C77.2 C78.2 C79.2 C80.2 ; also sheet 1,2,4
VBN: C5.1 C10.1 C15.1 C20.1 C25.1 C30.1 C35.1 C40.1 C45.1 C50.1 C55.1 C60.1 C65.1 C70.1 C75.1 C80.1 ; also sheet 1,2,4
VBP: C4.1 C9.1 C14.1 C19.1 C24.1 C29.1 C34.1 C39.1 C44.1 C49.1 C54.1 C59.1 C64.1 C69.1 C74.1 C79.1 ; also sheet 1,2,4
VCCQ: C3.1 C8.1 C13.1 C18.1 C23.1 C28.1 C33.1 C38.1 C43.1 C48.1 C53.1 C58.1 C63.1 C68.1 C73.1 C78.1 ; also sheet 1,2,4
VDD: C1.1 C2.1 C6.1 C7.1 C11.1 C12.1 C16.1 C17.1 C21.1 C22.1 C26.1 C27.1 C31.1 C32.1 C36.1 C37.1 C41.1 C42.1 C46.1 C47.1 C51.1 C52.1 C56.1 C57.1 C61.1 C62.1 C66.1 C67.1 C71.1 C72.1 C76.1 C77.1 ; also sheet 1,2,4

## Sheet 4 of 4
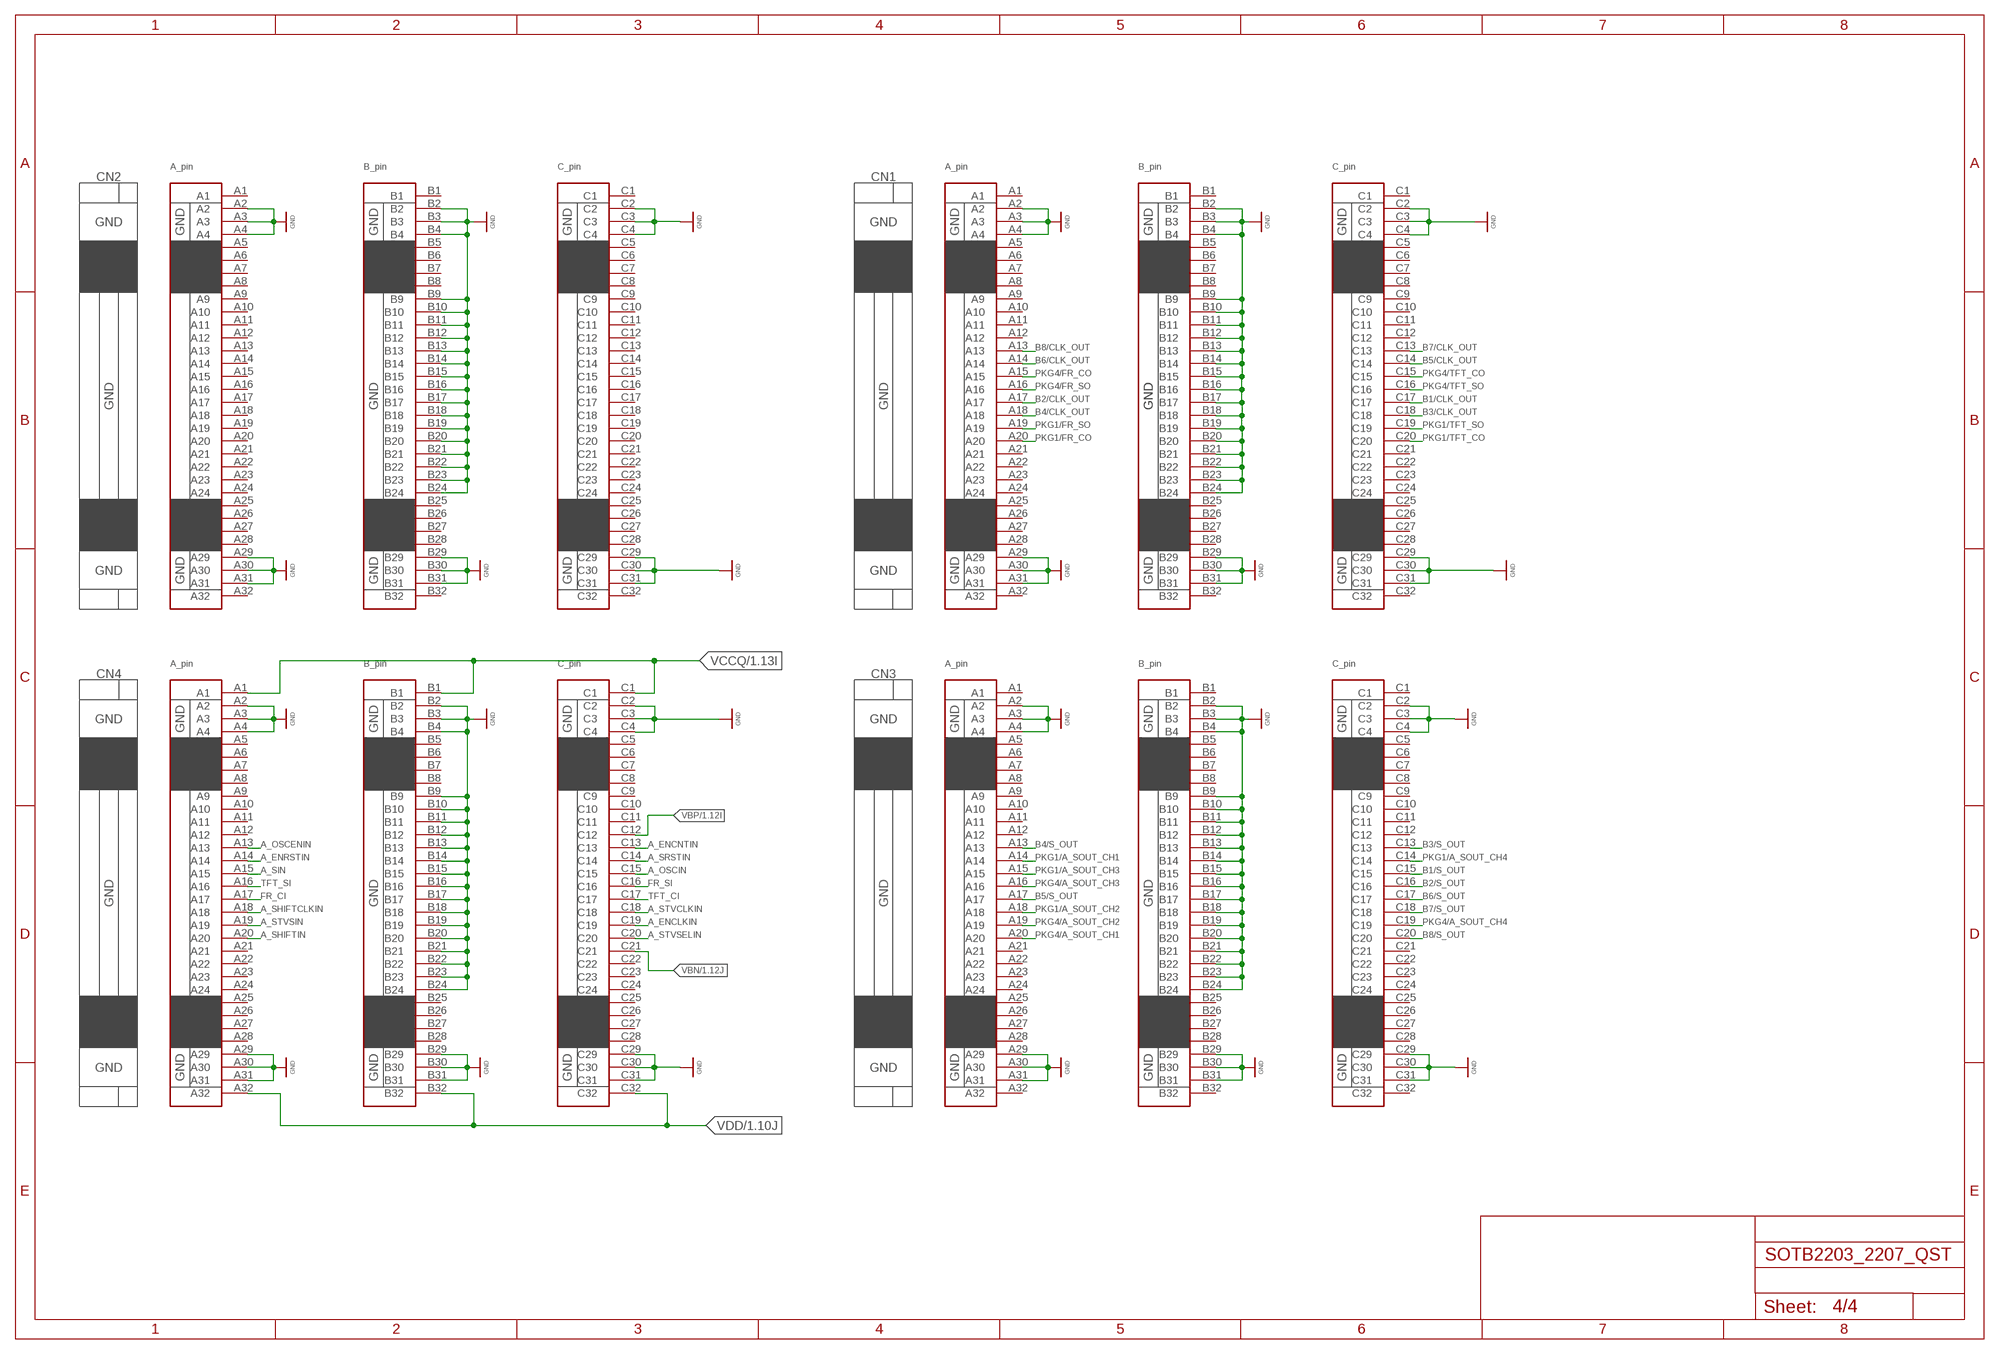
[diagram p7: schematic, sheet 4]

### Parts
CN5  XC5G-9621  [XC5D_9623]
CN6  XC5G-9621  [XC5D_9623]
CN7  XC5G-9621  [XC5D_9623]
CN8  XC5G-9621  [XC5D_9623]

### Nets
A_ENCLKIN: CN8.C19 ; also sheet 1,2
A_ENCNTIN: CN8.C13 ; also sheet 1,2
A_ENRSTIN: CN8.A14 ; also sheet 1,2
A_OSCENIN: CN8.A13 ; also sheet 1,2
A_OSCIN: CN8.C15 ; also sheet 1,2
A_SHIFTCLKIN: CN8.A18 ; also sheet 1,2
A_SHIFTIN: CN8.A20 ; also sheet 1,2
A_SIN: CN8.A15 ; also sheet 1,2
A_SRSTIN: CN8.C14 ; also sheet 1,2
A_STVCLKIN: CN8.C18 ; also sheet 1,2
A_STVSELIN: CN8.C20 ; also sheet 1,2
A_STVSIN: CN8.A19 ; also sheet 1,2
B1/CLK_OUT: CN5.C17 ; also sheet 1,2
B1/S_OUT: CN7.C15 ; also sheet 1,2
B2/CLK_OUT: CN5.A17 ; also sheet 1,2
B2/S_OUT: CN7.C16 ; also sheet 1,2
B3/CLK_OUT: CN5.C18 ; also sheet 1,2
B3/S_OUT: CN7.C13 ; also sheet 1,2
B4/CLK_OUT: CN5.A18 ; also sheet 1,2
B4/S_OUT: CN7.A13 ; also sheet 1,2
B5/CLK_OUT: CN5.C14 ; also sheet 1,2
B5/S_OUT: CN7.A17 ; also sheet 1,2
B6/CLK_OUT: CN5.A14 ; also sheet 1,2
B6/S_OUT: CN7.C17 ; also sheet 1,2
B7/CLK_OUT: CN5.C13 ; also sheet 1,2
B7/S_OUT: CN7.C18 ; also sheet 1,2
B8/CLK_OUT: CN5.A13 ; also sheet 1,2
B8/S_OUT: CN7.C20 ; also sheet 1,2
FR_CI: CN8.A17 ; also sheet 1,2
FR_SI: CN8.C16 ; also sheet 1,2
GND: CN5.A2 CN5.A3 CN5.A4 CN5.A29 CN5.A30 CN5.A31 CN5.B2 CN5.B3 CN5.B4 CN5.B9 CN5.B10 CN5.B11 CN5.B12 CN5.B13 CN5.B14 CN5.B15 CN5.B16 CN5.B17 CN5.B18 CN5.B19 CN5.B20 CN5.B21 CN5.B22 CN5.B23 CN5.B24 CN5.B29 CN5.B30 CN5.B31 CN5.C2 CN5.C3 CN5.C4 CN5.C29 CN5.C30 CN5.C31 CN6.A2 CN6.A3 CN6.A4 CN6.A29 CN6.A30 CN6.A31 CN6.B2 CN6.B3 CN6.B4 CN6.B9 CN6.B10 CN6.B11 CN6.B12 CN6.B13 CN6.B14 CN6.B15 CN6.B16 CN6.B17 CN6.B18 CN6.B19 CN6.B20 CN6.B21 CN6.B22 CN6.B23 CN6.B24 CN6.B29 CN6.B30 CN6.B31 CN6.C2 CN6.C3 CN6.C4 CN6.C29 CN6.C30 CN6.C31 CN7.A2 CN7.A3 CN7.A4 CN7.A29 CN7.A30 CN7.A31 CN7.B2 CN7.B3 CN7.B4 CN7.B9 CN7.B10 CN7.B11 CN7.B12 CN7.B13 CN7.B14 CN7.B15 CN7.B16 CN7.B17 CN7.B18 CN7.B19 CN7.B20 CN7.B21 CN7.B22 CN7.B23 CN7.B24 CN7.B29 CN7.B30 CN7.B31 CN7.C2 CN7.C3 CN7.C4 CN7.C29 CN7.C30 CN7.C31 CN8.A2 CN8.A3 CN8.A4 CN8.A29 CN8.A30 CN8.A31 CN8.B2 CN8.B3 CN8.B4 CN8.B9 CN8.B10 CN8.B11 CN8.B12 CN8.B13 CN8.B14 CN8.B15 CN8.B16 CN8.B17 CN8.B18 CN8.B19 CN8.B20 CN8.B21 CN8.B22 CN8.B23 CN8.B24 CN8.B29 CN8.B30 CN8.B31 CN8.C2 CN8.C3 CN8.C4 CN8.C29 CN8.C30 CN8.C31 ; also sheet 1,2,3
PKG1/A_SOUT_CH1: CN7.A14 ; also sheet 1,2
PKG1/A_SOUT_CH2: CN7.A18 ; also sheet 1,2
PKG1/A_SOUT_CH3: CN7.A15 ; also sheet 1,2
PKG1/A_SOUT_CH4: CN7.C14 ; also sheet 1,2
PKG1/FR_CO: CN5.A20 ; also sheet 1,2
PKG1/FR_SO: CN5.A19 ; also sheet 1,2
PKG1/TFT_CO: CN5.C20 ; also sheet 1,2
PKG1/TFT_SO: CN5.C19 ; also sheet 1,2
PKG4/A_SOUT_CH1: CN7.A20 ; also sheet 1,2
PKG4/A_SOUT_CH2: CN7.A19 ; also sheet 1,2
PKG4/A_SOUT_CH3: CN7.A16 ; also sheet 1,2
PKG4/A_SOUT_CH4: CN7.C19 ; also sheet 1,2
PKG4/FR_CO: CN5.A15 ; also sheet 1,2
PKG4/FR_SO: CN5.A16 ; also sheet 1,2
PKG4/TFT_CO: CN5.C15 ; also sheet 1,2
PKG4/TFT_SO: CN5.C16 ; also sheet 1,2
TFT_CI: CN8.C17 ; also sheet 1,2
TFT_SI: CN8.A16 ; also sheet 1,2
VBN: CN8.C21 ; also sheet 1,2,3
VBP: CN8.C12 ; also sheet 1,2,3
VCCQ: CN8.A1 CN8.B1 CN8.C1 ; also sheet 1,2,3
VDD: CN8.A32 CN8.B32 CN8.C32 ; also sheet 1,2,3
Unconnected: CN5.A1 CN5.A5 CN5.A6 CN5.A7 CN5.A8 CN5.A9 CN5.A10 CN5.A11 CN5.A12 CN5.A21 CN5.A22 CN5.A23 CN5.A24 CN5.A25 CN5.A26 CN5.A27 CN5.A28 CN5.A32 CN5.B1 CN5.B5 CN5.B6 CN5.B7 CN5.B8 CN5.B25 CN5.B26 CN5.B27 CN5.B28 CN5.B32 CN5.C1 CN5.C5 CN5.C6 CN5.C7 CN5.C8 CN5.C9 CN5.C10 CN5.C11 CN5.C12 CN5.C21 CN5.C22 CN5.C23 CN5.C24 CN5.C25 CN5.C26 CN5.C27 CN5.C28 CN5.C32 CN6.A1 CN6.A5 CN6.A6 CN6.A7 CN6.A8 CN6.A9 CN6.A10 CN6.A11 CN6.A12 CN6.A13 CN6.A14 CN6.A15 CN6.A16 CN6.A17 CN6.A18 CN6.A19 CN6.A20 CN6.A21 CN6.A22 CN6.A23 CN6.A24 CN6.A25 CN6.A26 CN6.A27 CN6.A28 CN6.A32 CN6.B1 CN6.B5 CN6.B6 CN6.B7 CN6.B8 CN6.B25 CN6.B26 CN6.B27 CN6.B28 CN6.B32 CN6.C1 CN6.C5 CN6.C6 CN6.C7 CN6.C8 CN6.C9 CN6.C10 CN6.C11 CN6.C12 CN6.C13 CN6.C14 CN6.C15 CN6.C16 CN6.C17 CN6.C18 CN6.C19 CN6.C20 CN6.C21 CN6.C22 CN6.C23 CN6.C24 CN6.C25 CN6.C26 CN6.C27 CN6.C28 CN6.C32 CN7.A1 CN7.A5 CN7.A6 CN7.A7 CN7.A8 CN7.A9 CN7.A10 CN7.A11 CN7.A12 CN7.A21 CN7.A22 CN7.A23 CN7.A24 CN7.A25 CN7.A26 CN7.A27 CN7.A28 CN7.A32 CN7.B1 CN7.B5 CN7.B6 CN7.B7 CN7.B8 CN7.B25 CN7.B26 CN7.B27 CN7.B28 CN7.B32 CN7.C1 CN7.C5 CN7.C6 CN7.C7 CN7.C8 CN7.C9 CN7.C10 CN7.C11 CN7.C12 CN7.C21 CN7.C22 CN7.C23 CN7.C24 CN7.C25 CN7.C26 CN7.C27 CN7.C28 CN7.C32 CN8.A5 CN8.A6 CN8.A7 CN8.A8 CN8.A9 CN8.A10 CN8.A11 CN8.A12 CN8.A21 CN8.A22 CN8.A23 CN8.A24 CN8.A25 CN8.A26 CN8.A27 CN8.A28 CN8.B5 CN8.B6 CN8.B7 CN8.B8 CN8.B25 CN8.B26 CN8.B27 CN8.B28 CN8.C5 CN8.C6 CN8.C7 CN8.C8 CN8.C9 CN8.C10 CN8.C11 CN8.C22 CN8.C23 CN8.C24 CN8.C25 CN8.C26 CN8.C27 CN8.C28

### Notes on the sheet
- CN2 | CN1
- GND | GND | GND | GND | GND | GND | GND | GND
- GND | GND | GND | GND | GND
- GND | GND | GND | GND | GND | GND | GND | GND
- CN4 | CN3
- GND | GND | GND | GND | GND | GND | GND | GND
- GND | GND | GND | GND
- GND | GND | GND | GND | GND | GND | GND | GND

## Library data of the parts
C1-C80 = rcl:C-EU: CAPACITOR, European symbol; SPICEPREFIX: C
CN1-CN8 = XC5G-9621:XC5G-9621
JP1-JP16 = pinhead:PINHD-1X5: PIN HEADER
PKG1 PKG4 = IC149-160:SOTB2207_4CHIP
U$5-U$8 = tantalum_capa_F93:TANTALUM_CAPA_F93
